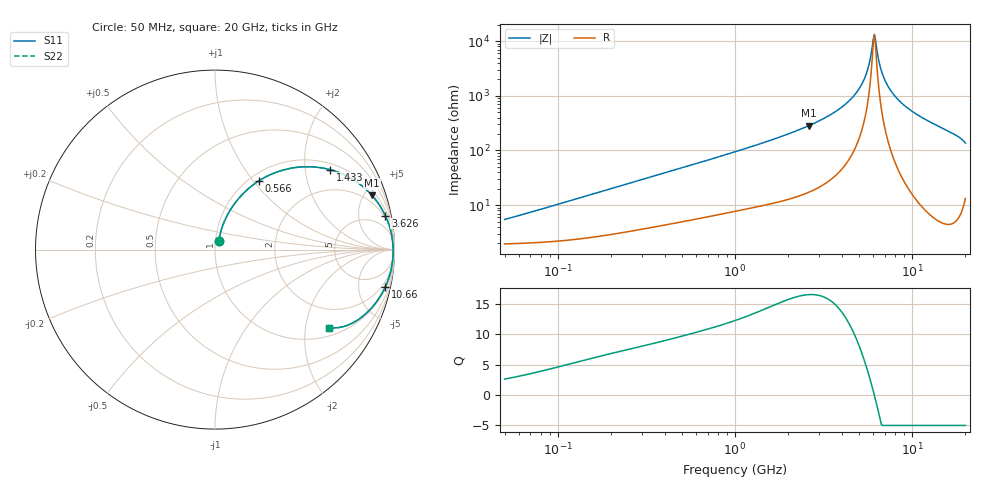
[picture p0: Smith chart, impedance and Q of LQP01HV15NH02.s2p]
!Murata Part Number: LQP01HV15NH02
!These Parameters are Measured in Series Mode Connection
!  o--[Z]--o
!Port1  Port2
!  o-------o
!Freq. Start=50[MHz] Stop=20[GHz], 401[Steps]
# Hz S RI R 50
!Freq.(Hz) S11(Real) S11(Imag) S21(Real) S21(Imag) S12(Real) S12(Imag) S22(Real) S22(Imag)
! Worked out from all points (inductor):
!   401 points, 50 MHz to 20 GHz, reference 50 ohm
!   read as one part in series: L = 16.2 nH near 58.96 MHz
!   highest Q = 16.5 at 2.608 GHz (marker M1), where L = 17.2 nH
!   self-resonance near 6.034 GHz
!   S11 on the Smith chart (normalised r, x): 50 MHz: 1.04, +0.10; 566 MHz: 1.11, +1.07; 1.433 GHz: 1.20, +2.73; 3.626 GHz: 1.66, +9.84; 10.66 GHz: 1.24, -9.06; 20 GHz: 1.26, -2.70
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5e7  0.0216 0.0489  0.9784 -0.0489  0.9784 -0.0489  0.0216 0.0489
1.364002e8  0.0409 0.1282  0.9591 -0.1282  0.9591 -0.1282  0.0409 0.1282
3.721004e8  0.1414 0.2956  0.8586 -0.2956  0.8586 -0.2956  0.1414 0.2956
5.659842e8  0.2461 0.3839  0.7539 -0.3839  0.7539 -0.3839  0.2461 0.3839
1e9  0.4728 0.46  0.5272 -0.46  0.5272 -0.46  0.4728 0.46
1.432596e9  0.6426 0.4448  0.3574 -0.4448  0.3574 -0.4448  0.6426 0.4448
2.608132e9  0.8748 0.302  0.1252 -0.302  0.1252 -0.302  0.8748 0.302
2.728004e9  0.8873 0.2874  0.1127 -0.2874  0.1127 -0.2874  0.8873 0.2874
3.626126e9  0.9489 0.1894  0.0511 -0.1894  0.0511 -0.1894  0.9489 0.1894
4.472136e9  0.9764 0.1141  0.0236 -0.1141  0.0236 -0.1141  0.9764 0.1141
5.117541e9  0.9868 0.0653  0.0132 -0.0653  0.0132 -0.0653  0.9868 0.0653
5.598765e9  0.9908 0.0325  0.0092 -0.0325  0.0092 -0.0325  0.9908 0.0325
5.944466e9  0.9922 0.0106  0.00782 -0.0106  0.00782 -0.0106  0.9922 0.0106
6.125241e9  0.9925 -0.000336  0.00751 0.000336  0.00751 0.000336  0.9925 -0.000336
6.311513e9  0.9925 -0.0113  0.00746 0.0113  0.00746 0.0113  0.9925 -0.0113
6.601595e9  0.9921 -0.0278  0.00786 0.0278  0.00786 0.0278  0.9921 -0.0278
6.802353e9  0.9916 -0.0389  0.00845 0.0389  0.00845 0.0389  0.9916 -0.0389
7.442007e9  0.9882 -0.0722  0.0118 0.0722  0.0118 0.0722  0.9882 -0.0722
8.644534e9  0.9771 -0.1282  0.0229 0.1282  0.0229 0.1282  0.9771 -0.1282
1.066139e10  0.9486 -0.2081  0.0514 0.2081  0.0514 0.2081  0.9486 -0.2081
1.621653e10  0.8247 -0.3703  0.1753 0.3703  0.1753 0.3703  0.8247 -0.3703
2e10  0.6357 -0.4349  0.3643 0.4349  0.3643 0.4349  0.6357 -0.4349
